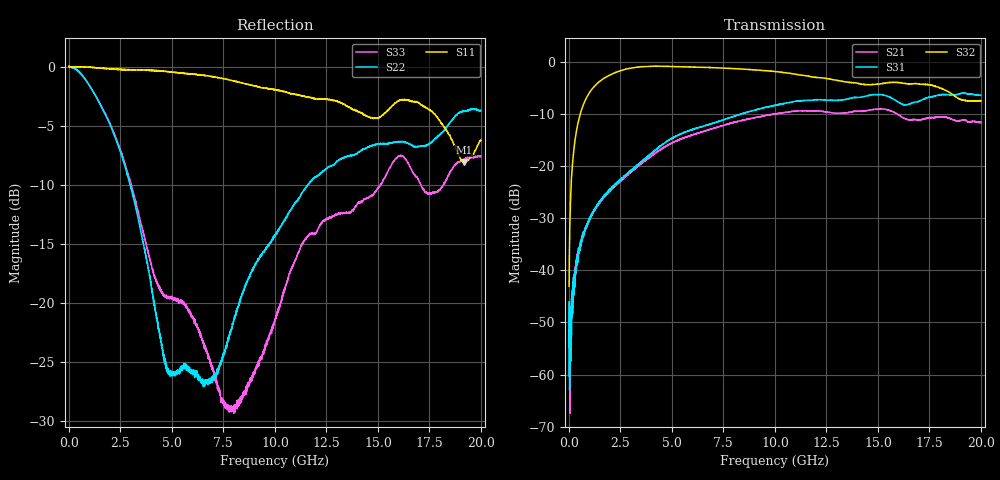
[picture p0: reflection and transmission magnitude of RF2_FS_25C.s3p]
!Keysight Technologies,N5244B,MY57181157,A.18.40.03
!Date: Friday, December 19, 2025 13:28:50
!Correction: S11(C  3-Port  )
!S12(C  3-Port  )
!S13(C  3-Port  )
!S21(C  3-Port  )
!S22(C  3-Port  )
!S23(C  3-Port  )
!S31(C  3-Port  )
!S32(C  3-Port  )
!S33(C  3-Port  )
!S3P File: Measurements: <S11,S12,S13>,
!<S21,S22,S23>,
!<S31,S32,S33>:
# Hz S  dB  R 50
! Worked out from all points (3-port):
!   3999 points, 10 MHz to 20 GHz, reference 50 ohm
!   strongest paths, dB at 10 MHz, 5.005 GHz, 10.01 GHz, 15.01 GHz, 20 GHz:
!     S32: -43.0, -0.9, -1.9, -4.3, -7.5
!     S31: -60.3, -14.7, -8.4, -6.3, -6.5
!     S21: -51.5, -15.6, -10.0, -9.1, -11.7
!   lowest |S11| = -8.1 dB at 19.16 GHz (marker M1), VSWR 2.30, Z = 22.4 + j7.79 ohm
!   |S11| at or under -10 dB: nowhere
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1e7  0.04 -0.3  -50.73 -72.0  -58.37 -169.2
     -51.46 175.8  0.01 -0.4  -44.36 115.0
     -60.27 -115.2  -43.05 77.0  0.04 -0.4
1.5e8  -0.01 -1.4  -48.98 88.5  -46.47 98.2
       -44.76 93.5  -0.05 -6.7  -21.02 86.1
       -45.37 98.4  -20.97 86.9  -0.06 -6.5
3.55e8  -0.02 -3.3  -39.36 90.6  -39.50 93.3
        -40.17 88.4  -0.23 -15.5  -13.59 75.5
        -39.59 93.2  -13.53 75.0  -0.24 -15.0
1.39e9  -0.10 -12.1  -27.55 77.1  -27.35 82.5
        -27.53 76.8  -2.78 -51.2  -4.15 37.5
        -27.40 82.3  -4.14 37.5  -2.74 -47.8
4.865e9  -0.41 -30.5  -15.86 52.8  -15.00 67.4
         -15.87 53.3  -25.94 -132.2  -0.93 -24.0
         -15.01 67.5  -0.93 -24.0  -19.53 -65.7
7.835e9  -1.14 -60.6  -11.83 20.5  -10.68 40.8
         -11.86 20.7  -22.43 108.8  -1.29 -55.1
         -10.71 41.0  -1.31 -55.2  -28.81 -87.6
1.0005e10  -1.95 -84.2  -10.01 -5.0  -8.38 20.5
           -10.02 -5.0  -14.32 98.8  -1.90 -76.5
           -8.37 20.5  -1.90 -76.5  -21.42 -142.9
1.6125e10  -2.80 -162.3  -10.52 -82.6  -8.08 -39.4
           -10.51 -82.7  -6.34 80.2  -4.08 -123.3
           -8.07 -39.2  -4.10 -123.1  -7.50 174.6
1.9165e10  -8.11 158.1  -11.18 -105.3  -6.03 -54.4
           -11.18 -105.4  -3.75 34.7  -7.38 -151.2
           -6.02 -54.4  -7.39 -151.2  -7.87 122.6
2e10  -6.24 148.6  -11.68 -113.9  -6.44 -61.1
      -11.66 -113.8  -3.71 45.2  -7.47 -149.7
      -6.46 -61.0  -7.50 -149.4  -7.60 130.1
